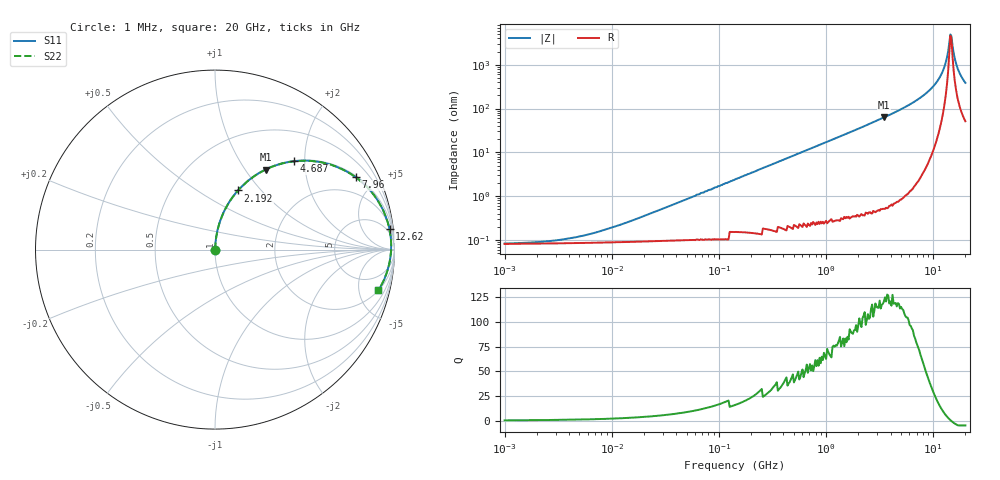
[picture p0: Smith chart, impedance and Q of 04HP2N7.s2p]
# MHz S MA R 50
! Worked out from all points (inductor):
!   431 points, 1 MHz to 20 GHz, reference 50 ohm
!   read as one part in series: L = 2.7 nH near 16.23 MHz
!   highest Q = 121 at 3.474 GHz (marker M1), where L = 2.86 nH
!   self-resonance near 14.49 GHz
!   S11 on the Smith chart (normalised r, x): 1 MHz: 1.00, +0.00; 2.192 GHz: 1.01, +0.76; 4.687 GHz: 1.01, +1.77; 7.96 GHz: 1.06, +3.84; 12.62 GHz: 3, +17; 20 GHz: 2.04, -7.66
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1  0.0006468 15.2  0.999 -0.0  0.999 -0.0  0.0006468 15.2
2.455  0.000781 32.2  0.999 -0.0  0.999 -0.0  0.000781 32.2
5.25  0.001137 51.5  0.999 -0.1  0.999 -0.1  0.001137 51.5
27.564  0.004758 78.8  0.999 -0.3  0.999 -0.3  0.004758 78.8
144.716  0.025 85.5  0.998 -1.4  0.998 -1.4  0.025 85.5
742.485  0.125 81.8  0.99 -7.2  0.99 -7.2  0.125 81.8
2191.796  0.354 68.7  0.932 -20.8  0.932 -20.8  0.354 68.7
3474.145  0.528 57.7  0.845 -31.9  0.845 -31.9  0.528 57.7
3898.162  0.578 54.2  0.811 -35.3  0.811 -35.3  0.578 54.2
4686.829  0.661 48.2  0.745 -41.3  0.745 -41.3  0.661 48.2
7960.387  0.881 27.3  0.459 -61.8  0.459 -61.8  0.881 27.3
10494.53  0.955 15.0  0.26 -72.6  0.26 -72.6  0.955 15.0
11775.38  0.972 9.8  0.171 -75.8  0.171 -75.8  0.972 9.8
12617.75  0.979 6.7  0.117 -76.1  0.117 -76.1  0.979 6.7
13212.56  0.981 4.6  0.081 -74.2  0.081 -74.2  0.981 4.6
14157.74  0.982 1.4  0.031 -53.3  0.031 -53.3  0.982 1.4
14825.14  0.981 -0.6  0.022 29.5  0.022 29.5  0.981 -0.6
15170.55  0.979 -1.7  0.036 53.9  0.036 53.9  0.979 -1.7
16255.8  0.974 -4.8  0.086 70.0  0.086 70.0  0.974 -4.8
17022.1  0.968 -6.8  0.122 71.5  0.122 71.5  0.968 -6.8
18664.78  0.953 -10.9  0.191 70.5  0.191 70.5  0.953 -10.9
20000  0.938 -13.9  0.243 68.5  0.243 68.5  0.938 -13.9
